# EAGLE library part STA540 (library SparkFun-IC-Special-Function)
Multiwatt package for L298 bridge driver
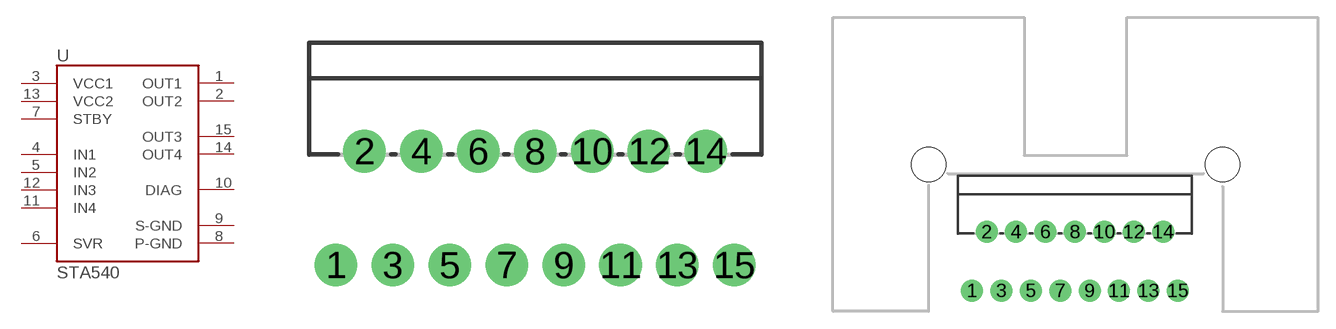
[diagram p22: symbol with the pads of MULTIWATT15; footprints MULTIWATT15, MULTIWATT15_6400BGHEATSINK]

Designator prefix -

## STA540  [MULTIWATT15]
1  OUT1
2  OUT2
3  VCC1
4  IN1
5  IN2
6  SVR
7  STBY
8  P-GND
9  S-GND
10  DIAG
11  IN4
12  IN3
13  VCC2
14  OUT4
15  OUT3

## STA540W/6400BG_HEATSINK  [MULTIWATT15_6400BGHEATSINK]
Pads as for MULTIWATT15

## STA540W/YB324G_HEATSINK  [MULTIWATT15_YB324GHEATSINK]
Pads as for MULTIWATT15

## STA5406400BG_W/SOLDERPOSTS  [MULTIWATT15_6400BGHEATSINK_2]
Pads as for MULTIWATT15

## Footprint MULTIWATT15 (pad centres in mm)
Multiwatt15V package for the L298 dual full bridge driver
drill 1.1 pad 1.9: 1 -8.95,-2.39; 2 -7.68,2.69; 3 -6.41,-2.39; 4 -5.14,2.69; 5 -3.87,-2.39; 6 -2.6,2.69; 7 -1.33,-2.39; 8 -0.06,2.69; 9 1.21,-2.39; 10 2.48,2.69; 11 3.75,-2.39; 12 5.02,2.69; 13 6.29,-2.39; 14 7.56,2.69; 15 8.83,-2.39

## Footprint MULTIWATT15_6400BGHEATSINK (pad centres in mm)
drill 1.1 pad 1.9: 1 -8.95,-2.39; 2 -7.68,2.69; 3 -6.41,-2.39; 4 -5.14,2.69; 5 -3.87,-2.39; 6 -2.6,2.69; 7 -1.33,-2.39; 8 -0.06,2.69; 9 1.21,-2.39; 10 2.48,2.69; 11 3.75,-2.39; 12 5.02,2.69; 13 6.29,-2.39; 14 7.56,2.69; 15 8.83,-2.39
hole 2.997 at -12.7,8.509
hole 2.997 at 12.7,8.509

## Footprint MULTIWATT15_YB324GHEATSINK (pad centres in mm)
drill 1.1 pad 1.9: 1 -8.95,-2.39; 2 -7.68,2.69; 3 -6.41,-2.39; 4 -5.14,2.69; 5 -3.87,-2.39; 6 -2.6,2.69; 7 -1.33,-2.39; 8 -0.06,2.69; 9 1.21,-2.39; 10 2.48,2.69; 11 3.75,-2.39; 12 5.02,2.69; 13 6.29,-2.39; 14 7.56,2.69; 15 8.83,-2.39
hole 2.997 at 19.152,4.445
hole 2.997 at -19.152,4.445

## Footprint MULTIWATT15_6400BGHEATSINK_2 (pad centres in mm)
drill 1.1 pad 1.9: 1 -8.95,-2.39; 2 -7.68,2.69; 3 -6.41,-2.39; 4 -5.14,2.69; 5 -3.87,-2.39; 6 -2.6,2.69; 7 -1.33,-2.39; 8 -0.06,2.69; 9 1.21,-2.39; 10 2.48,2.69; 11 3.75,-2.39; 12 5.02,2.69; 13 6.29,-2.39; 14 7.56,2.69; 15 8.83,-2.39
drill 2.413 pad 3.81: P$1 -12.7,8.509; P$2 12.7,8.509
